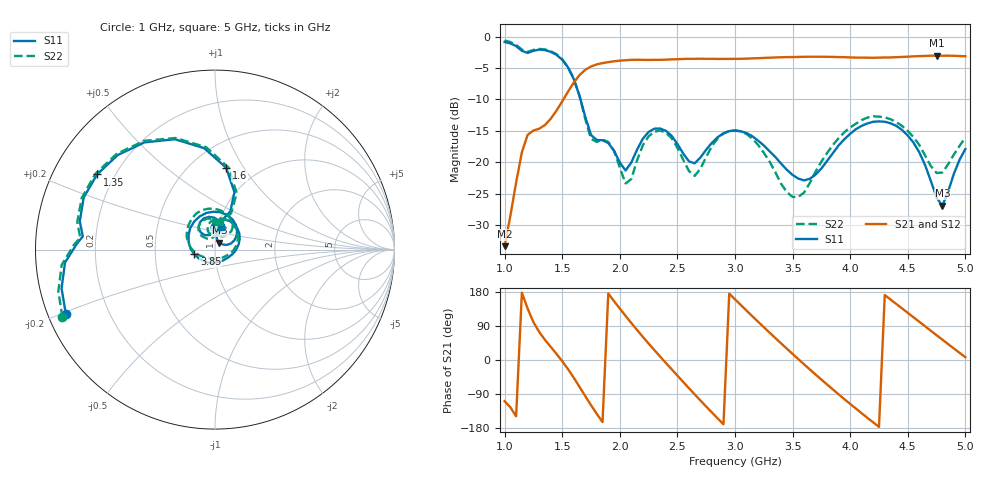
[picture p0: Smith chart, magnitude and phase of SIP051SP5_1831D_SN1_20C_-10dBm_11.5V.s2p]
# GHz  S  dB  R  50
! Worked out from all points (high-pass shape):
!   81 points, 1 GHz to 5 GHz, reference 50 ohm
!   highest |S21| = -3.04 dB at 4.75 GHz (marker M1); lowest = -33.3 dB at 1 GHz (marker M2)
!   |S21| within 3 dB of the highest: 1.656 GHz to end of sweep
!   lowest |S11| = -26.9 dB at 4.8 GHz (marker M3), VSWR 1.09, Z = 52.4 + j3.97 ohm
!   |S11| at or under -10 dB: 1.659 GHz to end of sweep
!   |S22| runs from -25.5 to -0.6 dB; largest |S21 - S12| = 0.0029
!   S11 on the Smith chart (normalised r, x): 1 GHz: 0.05, -0.21; 1.35 GHz: 0.13, +0.29; 1.6 GHz: 0.72, +0.84; 3.85 GHz: 0.79, -0.04; 5 GHz: 1.03, +0.26
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1  -0.87 -156.7  -33.33 -108.7  -33.38 -107.3  -0.63 -156.0
1.2  -2.61 174.3  -15.63 135.6  -15.64 135.6  -2.46 174.9
1.35  -2.17 147.5  -14.08 53.4  -14.06 53.4  -2.06 147.6
1.6  -6.74 82.2  -7.34 -46.6  -7.34 -46.6  -6.70 80.6
1.7  -12.78 68.1  -5.30 -95.3  -5.31 -95.2  -13.10 66.1
1.85  -16.49 92.9  -4.23 -163.8  -4.23 -163.8  -16.39 93.6
1.95  -18.16 89.7  -3.94 155.3  -3.95 155.3  -18.18 84.8
2.05  -21.31 109.5  -3.78 116.4  -3.78 116.5  -23.36 99.9
2.15  -17.99 129.9  -3.70 79.1  -3.70 79.1  -19.67 134.6
2.35  -14.62 100.2  -3.71 9.1  -3.71 9.1  -14.97 104.1
2.65  -20.16 90.7  -3.55 -90.6  -3.54 -90.7  -22.17 93.8
2.85  -16.01 88.5  -3.56 -154.3  -3.57 -154.1  -16.20 100.5
3  -14.93 62.1  -3.55 160.1  -3.55 160.2  -14.97 70.1
3.3  -18.25 3.8  -3.36 72.2  -3.37 72.3  -19.88 -3.5
3.5  -22.02 -41.0  -3.27 16.0  -3.26 15.9  -25.51 -78.7
3.7  -21.94 -114.4  -3.22 -38.4  -3.22 -38.4  -21.46 -153.8
3.85  -18.54 -167.4  -3.24 -77.8  -3.24 -77.9  -17.24 174.6
4.1  -14.20 126.2  -3.36 -140.6  -3.35 -140.7  -13.28 126.0
4.35  -13.79 70.8  -3.33 159.6  -3.33 159.6  -13.14 81.3
4.75  -25.60 32.5  -3.04 65.4  -3.05 65.4  -21.70 63.3
4.8  -26.89 56.8  -3.06 53.7  -3.05 53.7  -21.62 76.0
5  -17.88 75.6  -3.13 7.3  -3.14 7.4  -16.08 78.8
